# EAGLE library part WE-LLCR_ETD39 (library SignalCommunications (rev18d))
WE-LLCR Resonant Converter Characteristics Transformer for high efficiency power supply Input voltage 360–400 VDC Switching frequency 70–120 kHz Output power 150 W–250 W Testing voltage 4 kVAC Litz wire for low eddy current losses Defined leakage inductance for use without additional resonant inductor Applications Power supplies for PC, netbook, LED lighting and other power supplies High efficient resonant converters Details see: http://katalog.we-online.de/en/pbs/WE-LLCR? Updated by Dan Xu 2014-07-07 2014 (C) Wurth Elektronik
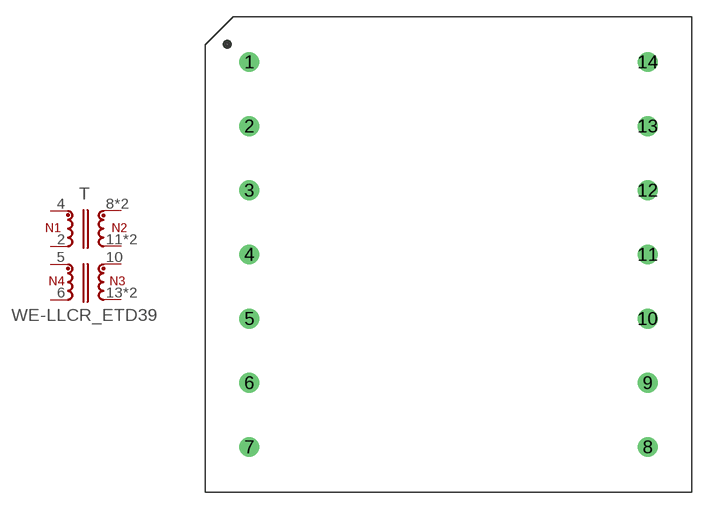
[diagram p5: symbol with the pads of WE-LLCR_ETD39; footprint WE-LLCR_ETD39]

Designator prefix T

## WE-LLCR_ETD39_760895631  [WE-LLCR_ETD39]
2  8  pas
4  1  pas
5  7  pas
6  6  pas
8  2  pas
9  2  pas
10  4  pas
11  3  pas
12  3  pas
13  5  pas
14  5  pas

## WE-LLCR_ETD39_760895641  [WE-LLCR_ETD39]
2  8  pas
4  1  pas
5  7  pas
6  6  pas
8  2  pas
10  4  pas
12  3  pas
14  5  pas

## WE-LLCR_ETD39_760895651  [WE-LLCR_ETD39]
Pads as for WE-LLCR_ETD39

## Footprint WE-LLCR_ETD39 (pad centres in mm)
size: ETD39 Height : 30mm max
drill 1.2: 1 -18,17.4; 2 -18,11.6; 3 -18,5.8; 4 -18,0; 5 -18,-5.8; 6 -18,-11.6; 7 -18,-17.4; 8 18,-17.4; 9 18,-11.6; 10 18,-5.8; 11 18,0; 12 18,5.8; 13 18,11.6; 14 18,17.4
